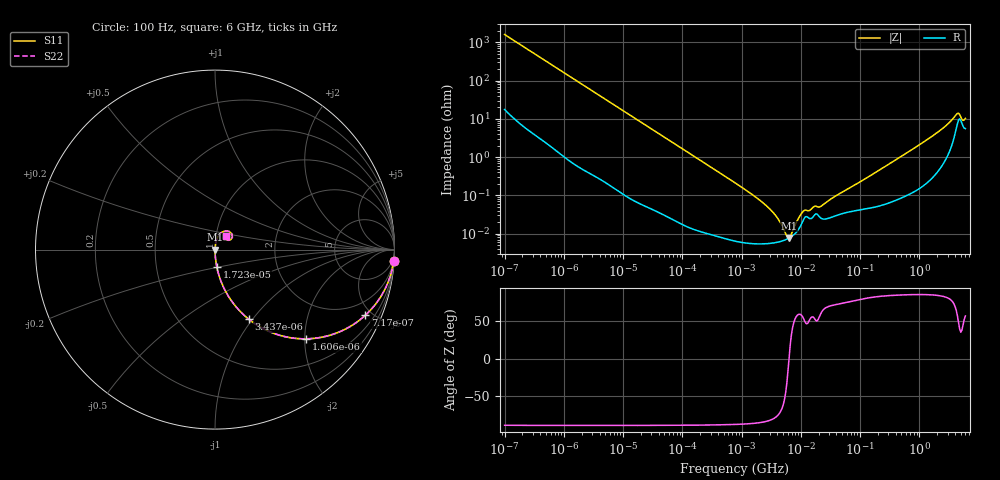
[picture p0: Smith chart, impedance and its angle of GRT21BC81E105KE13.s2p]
!Murata Part Number: GRT21BC81E105KE13
!These Parameters are Measured in Series Mode Connection
!Data Generated on Jun 19, 2026
!  o--ll--o
!Port1  Port2
!  o------o
!Operation Temp=25[degC], DC Bias Voltage=0[V]
!Freq. Start=100[Hz] Stop=6[GHz] 401[Steps]
# Hz S RI R 50
!Freq.(Hz) S11(Real) S11(Imag) S21(Real) S21(Imag) S12(Real) S12(Imag) S22(Real) S22(Imag)
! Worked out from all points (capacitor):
!   401 points, 100 Hz to 6 GHz, reference 50 ohm
!   read as one part in series: C = 982 nF near 109 Hz
!   lowest |Z| = 7.72 mohm at 6.353 MHz (marker M1)
!   series resonance near 6.32 MHz, so ESL is about 650 pH
!   S11 on the Smith chart (normalised r, x): 100 Hz: 1, -32; 717 Hz: 1.03, -4.55; 1.606 kHz: 1.01, -2.04; 3.437 kHz: 1.01, -0.95; 17.23 kHz: 1.00, -0.19; 6 GHz: 1.11, +0.17
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100  0.9955 -0.0614  0.00446 0.0614  0.00446 0.0614  0.9955 -0.0614
335  0.9579 -0.197  0.0421 0.197  0.0421 0.197  0.9579 -0.197
717  0.8364 -0.3665  0.1636 0.3665  0.1636 0.3665  0.8364 -0.3665
1606  0.5093 -0.4969  0.4907 0.4969  0.4907 0.4969  0.5093 -0.4969
2008  0.3998 -0.4868  0.6002 0.4868  0.6002 0.4868  0.3998 -0.4868
3437  0.1871 -0.3868  0.8129 0.3868  0.8129 0.3868  0.1871 -0.3868
6728  0.0578 -0.23  0.9422 0.23  0.9422 0.23  0.0578 -0.23
17227  0.00974 -0.0948  0.9903 0.0948  0.9903 0.0948  0.00974 -0.0948
40335  0.00204 -0.041  0.998 0.041  0.998 0.041  0.00204 -0.041
774597  6.84e-05 -0.00214  0.9999 0.00214  0.9999 0.00214  6.84e-05 -0.00214
2837864  5.54e-05 -0.000478  0.9999 0.000478  0.9999 0.000478  5.54e-05 -0.000478
4060267  6e-05 -0.000247  0.9999 0.000247  0.9999 0.000247  6e-05 -0.000247
5554849  6.97e-05 -7.08e-05  0.9999 7.08e-05  0.9999 7.08e-05  6.97e-05 -7.08e-05
6353432  7.71e-05 3e-06  0.9999 -3e-06  0.9999 -3e-06  7.71e-05 3e-06
7266822  8.83e-05 7.84e-05  0.9999 -7.84e-05  0.9999 -7.84e-05  8.83e-05 7.84e-05
1.087309e7  0.000217 0.000313  0.9998 -0.000313  0.9998 -0.000313  0.000217 0.000313
1.555665e7  0.000259 0.000385  0.9997 -0.000385  0.9997 -0.000385  0.000259 0.000385
2.225763e7  0.00025 0.000469  0.9998 -0.000469  0.9998 -0.000469  0.00025 0.000469
3.124326e8  0.000686 0.00667  0.9993 -0.00667  0.9993 -0.00667  0.000686 0.00667
1.873145e9  0.00514 0.0403  0.9949 -0.0403  0.9949 -0.0403  0.00514 0.0403
4.193612e9  0.0632 0.1044  0.9368 -0.1044  0.9368 -0.1044  0.0632 0.1044
6e9  0.0595 0.0775  0.9405 -0.0775  0.9405 -0.0775  0.0595 0.0775
